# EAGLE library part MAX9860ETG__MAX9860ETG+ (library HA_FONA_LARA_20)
Audio Codec 1ADC / 2DAC 16-Bit 24-Pin TQFN EP
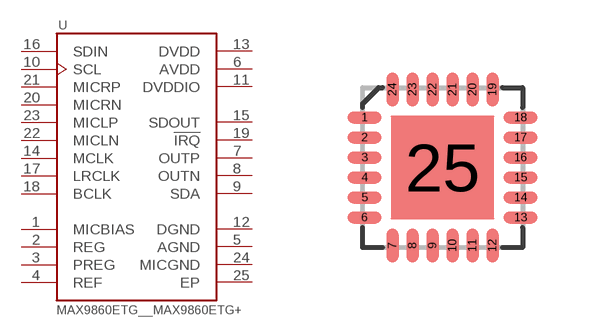
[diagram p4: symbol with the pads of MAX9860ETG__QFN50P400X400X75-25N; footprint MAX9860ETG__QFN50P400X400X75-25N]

Designator prefix U

## MAX9860ETG__MAX9860ETG+ (AVAILABILITY: Unavailable; DESCRIPTION: Audio Interface 16 b Serial 24-TQFN (4x4); MF: Maxim Integrated; MP: MAX9860ETG+; PACKAGE: TQFN-24 Maxim; PRICE: None)  [MAX9860ETG__QFN50P400X400X75-25N]
1  MICBIAS  pas
2  REG  pas
3  PREG  pas
4  REF  pas
5  AGND  pwr
6  AVDD  pwr
7  OUTP  out
8  OUTN  out
9  SDA  out
10  SCL  in
11  DVDDIO  pwr
12  DGND  pwr
13  DVDD  pwr
14  MCLK  in
15  SDOUT  out
16  SDIN  in
17  LRCLK
18  BCLK
19  !IRQ  out
20  MICRN  in
21  MICRP  in
22  MICLN  in
23  MICLP  in
24  MICGND  pwr
25  EP  pwr

## Footprint MAX9860ETG__QFN50P400X400X75-25N (pad centres in mm)
smd 0.85 x 0.3: 1 -1.95,1.25; 2 -1.95,0.75; 3 -1.95,0.25; 4 -1.95,-0.25; 5 -1.95,-0.75; 6 -1.95,-1.25; 13 1.95,-1.25; 14 1.95,-0.75; 15 1.95,-0.25; 16 1.95,0.25; 17 1.95,0.75; 18 1.95,1.25
smd 0.3 x 0.85: 7 -1.25,-1.95; 8 -0.75,-1.95; 9 -0.25,-1.95; 10 0.25,-1.95; 11 0.75,-1.95; 12 1.25,-1.95; 19 1.25,1.95; 20 0.75,1.95; 21 0.25,1.95; 22 -0.25,1.95; 23 -0.75,1.95; 24 -1.25,1.95
smd 2.6 x 2.6: 25 0,0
